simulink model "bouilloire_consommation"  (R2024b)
settings: Solver=VariableStepAuto  StartTime=0.0  StopTime=300  RelTol=1e-3  EnableMultiTasking=on
libraries: fl_lib x11, nesl_utility x4, slpidlib x1

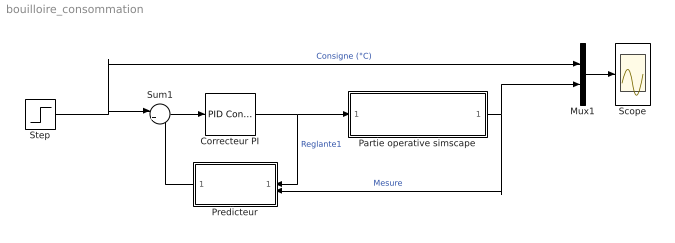
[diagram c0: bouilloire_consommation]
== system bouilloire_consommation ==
  Correcteur PI : slpidlib/PID Controller  Controller=PI  Form=Parallel  TimeDomain=Continuous-time  UseExternalTs=off  SampleTime=-1  IntegratorMethod=Forward Euler  FilterMethod=Forward Euler  ControllerParametersSource=internal  P=100  I=0.0026  UseKiTs=off  D=0.1  UseExternalDerivativeSource=off  N=50  UseFilter=on  TunerSelectOption=Transfer Function Based (PID Tuner App)  InitialConditionSource=internal  InitialConditionForIntegrator=0  InitialConditionForFilter=0  DifferentiatorICPrevScaledInput=0  ExternalReset=none  TrackingMode=off  Kt=1  LimitOutput=on  SatLimitsSource=internal  UpperSaturationLimit=100  LowerSaturationLimit=0  LinearizeAsGain=off  AntiWindupMode=back-calculation  Kb=0.0001  LimitIntegrator=off  UpperIntegratorSaturationLimit=inf  LowerIntegratorSaturationLimit=-inf  PGainOutDataTypeStr=double  PProdOutDataTypeStr=double  POutMin=[]  POutMax=[]  IGainOutDataTypeStr=double  IProdOutDataTypeStr=double  IOutMin=[]  IOutMax=[]  DGainOutDataTypeStr=double  DProdOutDataTypeStr=double  DOutMin=[]  DOutMax=[]  NGainOutDataTypeStr=double  NProdOutDataTypeStr=double  NOutMin=[]  NOutMax=[]  SumOutDataTypeStr=double  SumOutMin=[]  SumOutMax=[]  SaturationOutMin=[]  SaturationOutMax=[]  PParamDataTypeStr=double  PParamMin=[]  PParamMax=[]  IParamDataTypeStr=double  IParamMin=[]  IParamMax=[]  DParamDataTypeStr=double  DParamMin=[]  DParamMax=[]  NParamDataTypeStr=double  NParamMin=[]  NParamMax=[]  KbParamMin=[]  KbParamMax=[]  KtParamMin=[]  KtParamMax=[]  KbOutMin=[]  KbOutMax=[]  KtOutMin=[]  KtOutMax=[]  IntegratorOutDataTypeStr=double  IntegratorOutMin=[]  IntegratorOutMax=[]  FilterOutDataTypeStr=double  FilterOutMin=[]  FilterOutMax=[]  SumI1OutMin=[]  SumI1OutMax=[]  SumI2OutMin=[]  SumI2OutMax=[]  SumI3OutMin=[]  SumI3OutMax=[]  SumI4OutMin=[]  SumI4OutMax=[]  SumDOutDataTypeStr=double  SumDOutMin=[]  SumDOutMax=[]  SumAccumDataTypeStr=double  SumDAccumDataTypeStr=double  DifferentiatorOutMin=[]  DifferentiatorOutMax=[]  FilterDiffOutCoefMin=[]  FilterDiffOutCoefMax=[]  ReciprocalOutMin=[]  ReciprocalOutMax=[]  SumDenOutMin=[]  SumDenOutMax=[]  SumNumOutMin=[]  SumNumOutMax=[]  DivideOutMin=[]  DivideOutMax=[]  UdiffTsProdOutMin=[]  UdiffTsProdOutMax=[]  NTsProdOutMin=[]  NTsProdOutMax=[]  UintegralTsProdOutMin=[]  UintegralTsProdOutMax=[]  UngainTsProdOutMin=[]  UngainTsProdOutMax=[]  ClampingZeroOutDataTypeStr=Inherit: Inherit via back propagation  ClampingZeroOutMin=[]  ClampingZeroOutMax=[]  FilterDenConstantOutDataTypeStr=Inherit: Inherit via back propagation  FilterDenConstantOutMin=[]  FilterDenConstantOutMax=[]  PCopyOutDataTypeStr=Inherit: Inherit via back propagation  PCopyOutMin=[]  PCopyOutMax=[]  NCopyOutDataTypeStr=Inherit: Inherit via back propagation  NCopyOutMin=[]  NCopyOutMax=[]  IntegratorContinuousStateAttributes=''  IntegratorStateMustResolveToSignalObject=off  IntegratorRTWStateStorageClass=Auto  FilterContinuousStateAttributes=''  FilterStateMustResolveToSignalObject=off  FilterRTWStateStorageClass=Auto  ParallelPVariant=InternalParameters  IdealPVariant=Disabled  IVariant=InternalParameters  DVariant=Disabled  IntegratorVariant=Continuous  SatVariant=Enabled  AWVariant=BackCalculation  PCopyVariant=Disabled  TRVariant=Disabled  FdbkBlocksVariant=Forward  IdealPFdbkVariant=Disabled  SatFdbkVariant=Disabled  DerivativeFilterVariant=Disabled  NVariant=Disabled  NCopyVariant=Disabled_SignalSpec  FilterICVariant=Disabled  IntegratorICVariant=InternalICs  ExternalResetVariant=Disabled  TRSumVariant=Passthrough  SumFdbkVariant=Disabled  SumVariant=Sum_PI  TsampFilterVariant=InternalTs  TsampNgainVariant=Passthrough  TsampIntegralVariant=Disabled_SignalSpec  ExternalSaturationOutDataTypeStr=Inherit: Same as second input  DerivativeSourceVariant=Disabled  PreIntVariant=InternalPreInt
  Mux1 : Mux  Inputs=2
  Partie operative simscape : Subsystem
  Predicteur : Subsystem
  Scope : Scope
  Step : Step  Before=20  After=30  SampleTime=0
  Sum1 : Sum  Inputs=|+-
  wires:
  Partie operative simscape/1(Out_temp_simul) -> Mux1/2, Predicteur/2(Temp (°C))  "Mesure"
  Step/1 -> Mux1/1, Sum1/1  "Consigne (°C)"
  Mux1/1 -> Scope/1
  Correcteur PI/1 -> Partie operative simscape/1(In_reglante), Predicteur/1(In1)  "Reglante1"
  Sum1/1 -> Correcteur PI/1
  Predicteur/1(Out1) -> Sum1/2

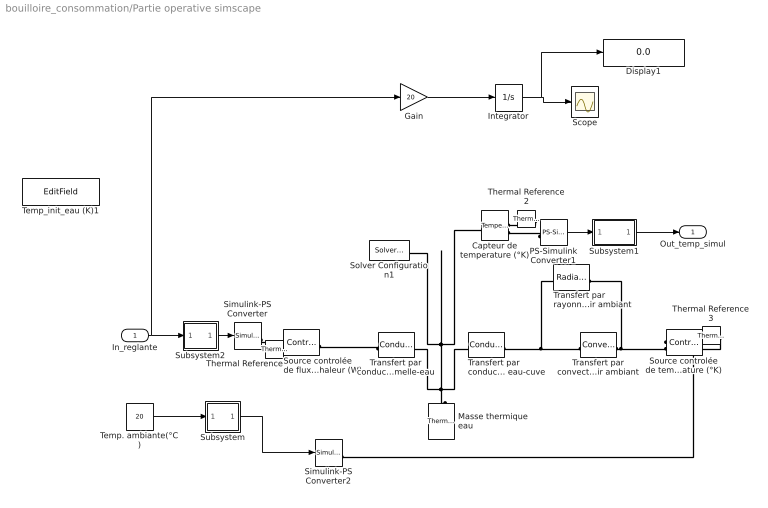
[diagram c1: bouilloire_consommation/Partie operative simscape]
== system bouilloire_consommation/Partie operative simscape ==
  In_reglante : Inport
  Capteur de temperature (°K) : fl_lib/Thermal/Thermal Sensors/Temperature Sensor  temperature_measure=foundation.enum.MeasurementReference.difference
  Display1 : Display
  Gain : Gain  Gain=20
  Integrator : Integrator
  Masse thermique eau : fl_lib/Thermal/Thermal Elements/Thermal Mass  mass_type=foundation.enum.constant_variable.constant  mass=0.5 kg  sp_heat=4180 J/kg/K  mass_min=1e-6 kg  num_ports=foundation.enum.numPorts2.one  m_specify=off  m_priority=High  m=1 kg  m_nominal_specify=off  m_nominal_value=1  m_nominal_unit=kg  T_specify=on  T_priority=High  T=293 K  T_nominal_specify=off  T_nominal_value=1  T_nominal_unit=K  Q_specify=on  Q_priority=None  Q=0 W  Q_nominal_specify=off  Q_nominal_value=1  Q_nominal_unit=W
  PS-Simulink Converter1 : nesl_utility/PS-Simulink Converter  PhysicalDomain=network_engine_domain  SubClassName=ps_output  LeftPortType=input  RightPortType=output  PseudoPeriodic=off  Frequencies=[]  VectorFormat=1-D array  Unit=1  AffineConversion=off
  Scope : Scope
  Simulink-PS Converter : nesl_utility/Simulink-PS Converter  PhysicalDomain=network_engine_domain  SubClassName=ps_input  LeftPortType=input  RightPortType=output  PseudoPeriodic=off  Frequencies=[]  NoiseDistribution=none  NoiseParameters=[]  Unit=1  AffineConversion=off  FilteringAndDerivatives=zero  SimscapeFilterOrder=1  InputFilterTimeConstant=0.001  UdotUserProvided=1
  Simulink-PS Converter2 : nesl_utility/Simulink-PS Converter  PhysicalDomain=network_engine_domain  SubClassName=ps_input  LeftPortType=input  RightPortType=output  PseudoPeriodic=off  Frequencies=[]  NoiseDistribution=none  NoiseParameters=[]  Unit=1  AffineConversion=off  FilteringAndDerivatives=zero  SimscapeFilterOrder=1  InputFilterTimeConstant=0.001  UdotUserProvided=1
  Solver Configuration1 : nesl_utility/Solver Configuration  PhysicalDomain=network_engine_domain  SubClassName=solver  LeftPortType=input  RightPortType=generic  Tones=[]  Harmonics=[]  SimulateNoise=off  Profile=off  UseLocalSampling=off  EnableSwitchedLinearOptims=on  FrequencyDomain=off  UseCCode=off  RelTol=0.001  AbsTol=1e-06  MinStep=1e-09  ToWorkspace=off  RevertToSquareIcSolve=off  NumHomotopyIterations=100  PhasorMode=off  PhasorModeNumHarmonics=1  ConsistencySolver=NEWTON_FTOL  IndexReductionMethod=DerivativeReplacement  DoDC=off  ResidualTolerance=1e-09  ConsistencyTolSource=GLOBAL  ConsistencyAbsTol=0.001  ConsistencyRelTol=0.001  ConsistencyTolFactor=0.001  UseLocalSolver=off  LocalSolverChoice=NE_BACKWARD_EULER_ADVANCER  ResolveIndetEquations=on  FunctionEvalNumThread=1  LocalSolverSampleTime=0.001  DoFixedCost=off  MaxNonlinIter=3  MaxModeIter=2  ComputeImpulses=off  ImpulseIterations=2  LinearAlgebra=Sparse  LinearAlgebraNumThread=0  EquationFormulation=NE_TIME_EF  DelaysMemoryBudget=1024  AutomaticFiltering=on  FilteringTimeConstant=0.001  PartitionStorageMethod=AS_NEEDED  PartitionMemoryBudget=1024  PartitionMethod=FAST  MultibodyUseLocalSolver=off  MultibodyLocalSolverChoice=ODE1  MultibodyLocalSolverSampleTime=0.001
  Source controlée de flux de chaleur (W) : fl_lib/Thermal/Thermal Sources/Controlled Heat Flow Rate Source
  Source controlée de temperature (°K) : fl_lib/Thermal/Thermal Sources/Controlled Temperature Source
  Subsystem : Subsystem
  Subsystem1 : Subsystem
  Subsystem2 : Subsystem
  Temp. ambiante(°C) : Constant  Value=20
  Temp_init_eau (K)1 : EditField  LabelPosition=Hide  ShowInitialText=on  Alignment=Center
  Thermal Reference : fl_lib/Thermal/Thermal Elements/Thermal Reference
  Thermal Reference2 : fl_lib/Thermal/Thermal Elements/Thermal Reference
  Thermal Reference3 : fl_lib/Thermal/Thermal Elements/Thermal Reference
  Transfert par rayonnement récipient-air ambiant : fl_lib/Thermal/Thermal Elements/Radiative Heat Transfer  area=61e-3 m^2  rad_tr_coeff=0.87*5.67e-8 W/(m^2*K^4)  T_specify=off  T_priority=None  T=0 K  T_nominal_specify=off  T_nominal_value=1  T_nominal_unit=K  Q_specify=off  Q_priority=None  Q=0 W  Q_nominal_specify=off  Q_nominal_value=1  Q_nominal_unit=W
  Transfert par conduction eau-cuve : fl_lib/Thermal/Thermal Elements/Conductive Heat Transfer  thermal_type=foundation.enum.ConstantVariableTabulated.Constant  wall_geometry=foundation.enum.ConductionWallGeometry.Planar  area=53e-3 m^2  thickness=0.9 mm  d_in=0.05 m  d_out=0.1 m  L=1 m  th_cond_min=10 W/(K*m)  th_cond=16 W/(m*K)  th_cond_TLU=[413, 401, 392, 383, 371, 357, 342] W/(K*m)  temp_TLU=[200, 273, 400, 600, 800, 1000, 1200] K  T_specify=off  T_priority=None  T=0 K  T_nominal_specify=off  T_nominal_value=1  T_nominal_unit=K  Q_specify=off  Q_priority=None  Q=0 W  Q_nominal_specify=off  Q_nominal_value=1  Q_nominal_unit=W
  Transfert par conduction semelle-eau : fl_lib/Thermal/Thermal Elements/Conductive Heat Transfer  thermal_type=foundation.enum.ConstantVariableTabulated.Constant  wall_geometry=foundation.enum.ConductionWallGeometry.Planar  area=13e-3 m^2  thickness=0.9 mm  d_in=0.05 m  d_out=0.1 m  L=1 m  th_cond_min=10 W/(K*m)  th_cond=16 W/(m*K)  th_cond_TLU=[413, 401, 392, 383, 371, 357, 342] W/(K*m)  temp_TLU=[200, 273, 400, 600, 800, 1000, 1200] K  T_specify=off  T_priority=None  T=0 K  T_nominal_specify=off  T_nominal_value=1  T_nominal_unit=K  Q_specify=off  Q_priority=None  Q=0 W  Q_nominal_specify=off  Q_nominal_value=1  Q_nominal_unit=W
  Transfert par convection cuve-air ambiant : fl_lib/Thermal/Thermal Elements/Convective Heat Transfer  thermal_type=foundation.enum.constant_variable.constant  area=61e-3 m^2  heat_tr_coeff=6.8 W/(m^2 * K)  min_heat_tr_coeff=1e-3 W/(K*m^2)  T_specify=off  T_priority=None  T=0 K  T_nominal_specify=off  T_nominal_value=1  T_nominal_unit=K  Q_specify=off  Q_priority=None  Q=0 W  Q_nominal_specify=off  Q_nominal_value=1  Q_nominal_unit=W
  Out_temp_simul : Outport  VectorParamsAs1DForOutWhenUnconnected=off
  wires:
  Temp. ambiante(°C)/1 -> Subsystem/1(E1)
  Subsystem/1(S1) -> Simulink-PS Converter2/1
  PS-Simulink Converter1/1 -> Subsystem1/1(E2)
  Subsystem1/1(S2) -> Out_temp_simul/1
  In_reglante/1 -> Gain/1, Subsystem2/1(E3)
  Subsystem2/1(S3) -> Simulink-PS Converter/1
  Integrator/1 -> Display1/1, Scope/1
  Gain/1 -> Integrator/1
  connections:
  Transfert par conduction semelle-eau/LConn1 -- Source controlée de flux de chaleur (W)/LConn1
  Transfert par rayonnement récipient-air ambiant/RConn1 -- Source controlée de temperature (°K)/LConn1 -- Transfert par convection cuve-air ambiant/RConn1
  Source controlée de temperature (°K)/RConn1 -- Simulink-PS Converter2/RConn1
  Thermal Reference2/LConn1 -- Capteur de temperature (°K)/RConn1
  Simulink-PS Converter/RConn1 -- Source controlée de flux de chaleur (W)/RConn1
  Thermal Reference/LConn1 -- Source controlée de flux de chaleur (W)/RConn2
  PS-Simulink Converter1/LConn1 -- Capteur de temperature (°K)/RConn2
  Thermal Reference3/LConn1 -- Source controlée de temperature (°K)/RConn2
  Transfert par convection cuve-air ambiant/LConn1 -- Transfert par rayonnement récipient-air ambiant/LConn1 -- Transfert par conduction eau-cuve/RConn1
  Masse thermique eau/LConn1 -- Solver Configuration1/RConn1 -- Capteur de temperature (°K)/LConn1 -- Transfert par conduction eau-cuve/LConn1 -- Transfert par conduction semelle-eau/RConn1

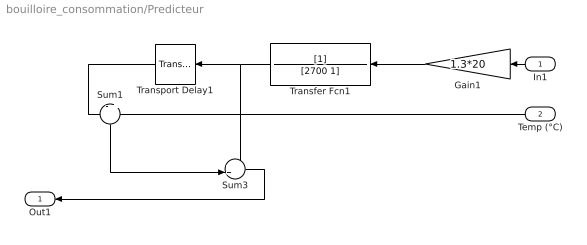
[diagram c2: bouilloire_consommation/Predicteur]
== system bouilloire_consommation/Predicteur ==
  In1 : Inport
  Temp (°C) : Inport  Port=2
  Gain1 : Gain  Gain=1.3*20
  Sum1 : Sum  Inputs=-|+
  Sum3 : Sum  Inputs=++|
  Transfer Fcn1 : TransferFcn  Denominator=[2700 1]
  Transport Delay1 : TransportDelay  DelayTime=26  BufferSize=2048
  Out1 : Outport  VectorParamsAs1DForOutWhenUnconnected=off
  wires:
  In1/1 -> Gain1/1
  Sum1/1 -> Sum3/2
  Transfer Fcn1/1 -> Sum3/1, Transport Delay1/1
  Sum3/1 -> Out1/1
  Gain1/1 -> Transfer Fcn1/1
  Temp (°C)/1 -> Sum1/2
  Transport Delay1/1 -> Sum1/1

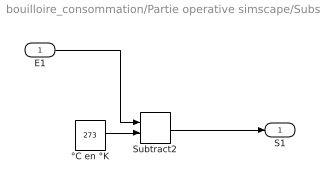
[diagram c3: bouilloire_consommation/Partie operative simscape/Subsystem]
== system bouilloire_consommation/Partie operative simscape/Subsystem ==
  E1 : Inport
  Subtract2 : Sum
  °C en °K : Constant  Value=273
  S1 : Outport  VectorParamsAs1DForOutWhenUnconnected=off
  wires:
  °C en °K/1 -> Subtract2/2
  Subtract2/1 -> S1/1
  E1/1 -> Subtract2/1

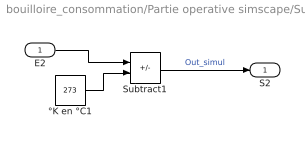
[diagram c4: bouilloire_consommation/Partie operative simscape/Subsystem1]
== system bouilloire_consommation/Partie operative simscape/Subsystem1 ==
  E2 : Inport
  Subtract1 : Sum  Inputs=+-
  °K en °C1 : Constant  Value=273
  S2 : Outport  VectorParamsAs1DForOutWhenUnconnected=off
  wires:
  °K en °C1/1 -> Subtract1/2
  E2/1 -> Subtract1/1
  Subtract1/1 -> S2/1  "Out_simul"

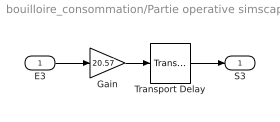
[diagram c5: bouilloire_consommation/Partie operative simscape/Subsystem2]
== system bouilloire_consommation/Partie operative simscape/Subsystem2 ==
  E3 : Inport
  Gain : Gain  Gain=20.57
  Transport Delay : TransportDelay  DelayTime=20  BufferSize=4096
  S3 : Outport  VectorParamsAs1DForOutWhenUnconnected=off
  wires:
  Gain/1 -> Transport Delay/1
  Transport Delay/1 -> S3/1
  E3/1 -> Gain/1
